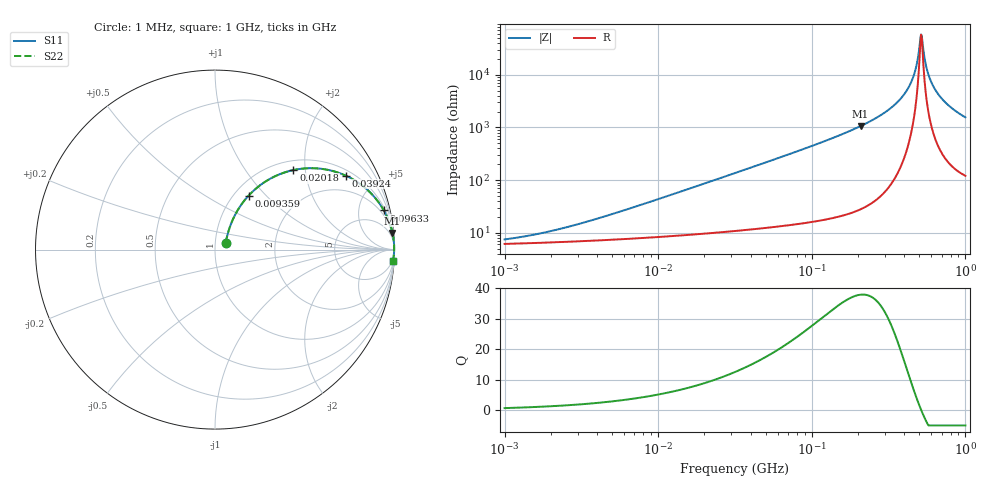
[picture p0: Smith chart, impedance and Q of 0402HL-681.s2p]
# MHz S MA R 50
!Freq  MagS11  AngS11  MagS21  AngS21  MagS12  AngS12  MagS22  AngS22
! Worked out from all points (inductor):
!   801 points, 1 MHz to 1 GHz, reference 50 ohm
!   read as one part in series: L = 680 nH near 5.248 MHz
!   highest Q = 37.9 at 207.7 MHz (marker M1), where L = 811 nH
!   self-resonance near 514.3 MHz
!   S11 on the Smith chart (normalised r, x): 1 MHz: 1.12, +0.09; 9.359 MHz: 1.16, +0.80; 20.18 MHz: 1.19, +1.73; 39.24 MHz: 1.23, +3.37; 96.33 MHz: 1.32, +8.53; 1 GHz: 3, -31
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1  0.07049 32.5  0.9413 -2.3  0.9413 -2.3  0.07049 32.5
3.180534  0.1415 55.7  0.9277 -7.2  0.9277 -7.2  0.1415 55.7
9.359443  0.354 58.1  0.8668 -20.3  0.8668 -20.3  0.354 58.1
10.02882  0.3748 57.4  0.8584 -21.6  0.8584 -21.6  0.3748 57.4
20.18366  0.6226 45.4  0.7164 -38.2  0.7164 -38.2  0.6226 45.4
31.89701  0.7794 34.5  0.5679 -51.0  0.5679 -51.0  0.7794 34.5
39.2419  0.8361 29.6  0.4947 -56.5  0.4947 -56.5  0.8361 29.6
96.32744  0.9657 13.1  0.2263 -74.8  0.2263 -74.8  0.9657 13.1
100.5773  0.9685 12.5  0.2167 -75.4  0.2167 -75.4  0.9685 12.5
207.7304  0.9931 5.4  0.09373 -83.1  0.09373 -83.1  0.9931 5.4
317.1393  0.9974 2.6  0.0458 -85.4  0.0458 -85.4  0.9974 2.6
383.4864  0.9982 1.6  0.02729 -85.4  0.02729 -85.4  0.9982 1.6
436.5158  0.9984 0.9  0.01528 -83.5  0.01528 -83.5  0.9984 0.9
471.7914  0.9984 0.5  0.008264 -78.6  0.008264 -78.6  0.9984 0.5
501.1872  0.9983 0.2  0.003108 -57.8  0.003108 -57.8  0.9983 0.2
514.3396  0.9983 0.0  0.001718 -9.7  0.001718 -9.7  0.9983 0.0
527.8372  0.9983 -0.1  0.002693 49.6  0.002693 49.6  0.9983 -0.1
551.1249  0.9982 -0.3  0.006237 72.6  0.006237 72.6  0.9982 -0.3
570.4926  0.998 -0.5  0.009295 77.6  0.009295 77.6  0.998 -0.5
632.776  0.9976 -1.1  0.0187 82.1  0.0187 82.1  0.9976 -1.1
765.156  0.9963 -2.1  0.03659 83.2  0.03659 83.2  0.9963 -2.1
1000  0.993 -3.7  0.06403 81.9  0.06403 81.9  0.993 -3.7
